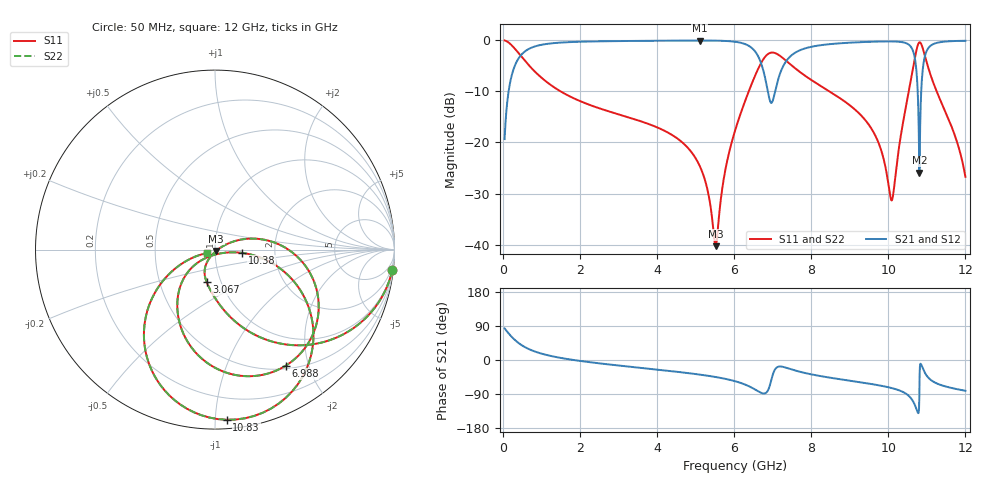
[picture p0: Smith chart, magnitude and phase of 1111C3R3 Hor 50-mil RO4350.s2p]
# GHz S MA R 50
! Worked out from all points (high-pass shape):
!   1601 points, 50 MHz to 12 GHz, reference 50 ohm
!   highest |S21| = -0.06 dB at 5.114 GHz (marker M1); lowest = -25.9 dB at 10.8 GHz (marker M2)
!   |S21| within 3 dB of the highest: 459.3 MHz to 6.62 GHz (6.16 GHz wide, 174 % of centre); 7.474 GHz to 10.68 GHz (3.203 GHz wide, 35.3 % of centre)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
!   lowest |S11| = -40.3 dB at 5.525 GHz (marker M3), VSWR 1.02, Z = 50.6 - j0.731 ohm
!   |S11| at or under -10 dB: 1.5 GHz to 6.382 GHz (4.882 GHz wide, 124 % of centre); 8.471 GHz to 10.53 GHz (2.061 GHz wide, 21.7 % of centre); 11.25 GHz to end of sweep
!   |S22| runs from -40.3 to -0.1 dB; largest |S21 - S12| = 0
!   S11 on the Smith chart (normalised r, x): 50 MHz: 1, -17; 3.067 GHz: 0.86, -0.32; 6.988 GHz: 0.54, -1.64; 10.38 GHz: 1.36, -0.05; 10.83 GHz: 0.05, -1.07; 12 GHz: 0.92, -0.03
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0.05  0.9942 -6.6  0.1079 83.4  0.1079 83.4  0.9942 -6.6
0.2217813  0.9013 -27.6  0.433 62.4  0.433 62.4  0.9013 -27.6
0.4831875  0.6933 -50.2  0.7201 39.7  0.7201 39.7  0.6933 -50.2
2.044156  0.2504 -92.7  0.9668 -2.9  0.9668 -2.9  0.2504 -92.7
3.067375  0.1853 -104.8  0.981 -15.2  0.981 -15.2  0.1853 -104.8
4.038312  0.1388 -114.8  0.9878 -25.7  0.9878 -25.7  0.1388 -114.8
5.113812  0.05853 -123.2  0.9925 -38.6  0.9925 -38.6  0.05853 -123.2
5.524594  0.009684 -48.1  0.99 -44.9  0.99 -44.9  0.009684 -48.1
6.025  0.13 22.7  0.9658 -55.9  0.9658 -55.9  0.13 22.7
6.532875  0.4381 -2.8  0.7877 -77.1  0.7877 -77.1  0.4381 -2.8
6.988469  0.7573 -58.7  0.2482 -44.4  0.2482 -44.4  0.7573 -58.7
7.39925  0.6073 -97.5  0.6576 -21.9  0.6576 -21.9  0.6073 -97.5
8.019156  0.4049 -121.0  0.8644 -38.2  0.8644 -38.2  0.4049 -121.0
9.483031  0.1514 -142.6  0.9634 -62.1  0.9634 -62.1  0.1514 -142.6
10.01331  0.03689 -116.5  0.9729 -72.1  0.9729 -72.1  0.03689 -116.5
10.12534  0.03063 -49.3  0.9719 -75.0  0.9719 -75.0  0.03063 -49.3
10.37928  0.1543 -6.9  0.9543 -84.3  0.9543 -84.3  0.1543 -6.9
10.66309  0.5893 -29.9  0.7391 -112.9  0.7391 -112.9  0.5893 -29.9
10.805  0.9522 -76.8  0.05078 -98.3  0.05078 -98.3  0.9522 -76.8
10.82741  0.9505 -86.0  0.1457 -11.6  0.1457 -11.6  0.9505 -86.0
11.03653  0.5395 -135.7  0.8351 -46.4  0.8351 -46.4  0.5395 -135.7
12  0.0461 -156.2  0.9866 -81.2  0.9866 -81.2  0.0461 -156.2
